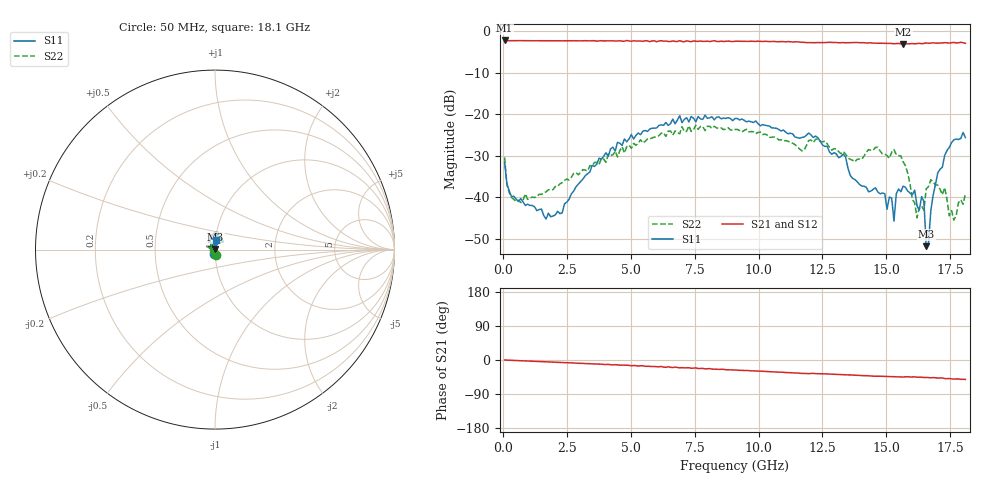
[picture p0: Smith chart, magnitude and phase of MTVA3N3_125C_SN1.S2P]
! Network Analyzer HP8720D.06.14 Serial No. US36140669
! 27 Jun 2005  08:55:49
! Frequency  S11  S21  S12  S22
# HZ  S  DB R 50
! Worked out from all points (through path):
!   201 points, 50 MHz to 18.1 GHz, reference 50 ohm
!   highest |S21| = -2.27 dB at 50 MHz (marker M1); lowest = -3.1 dB at 15.66 GHz (marker M2)
!   group delay of S21, straight-line fit = 7.91 ps
!   lowest |S11| = -51.8 dB at 16.57 GHz (marker M3), VSWR 1.01, Z = 50.2 + j0.173 ohm
!   |S11| at or under -10 dB: start of sweep to end of sweep
!   |S22| runs from -45.5 to -22.7 dB; largest |S21 - S12| = 0.022
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5e7  -31.66 -100.6  -2.27 0.1  -2.29 0.3  -30.42 -79.3
1.4025e8  -36.78 -122.5  -2.32 -0.3  -2.32 -0.2  -36.95 -115.0
5.0125e8  -40.44 -155.0  -2.33 -1.5  -2.32 -1.5  -41.04 -155.6
1.6745e9  -45.24 147.2  -2.34 -4.8  -2.34 -4.9  -38.70 161.6
3.1185e9  -35.62 79.8  -2.35 -8.9  -2.37 -9.1  -33.35 131.8
6.09675e9  -22.70 79.9  -2.41 -17.8  -2.35 -17.7  -25.16 79.4
9.075e9  -21.05 95.4  -2.47 -26.4  -2.45 -26.5  -23.70 51.4
1.21435e10  -25.63 125.2  -2.81 -35.3  -2.78 -35.5  -26.84 89.1
1.331675e10  -29.61 126.7  -2.79 -38.7  -2.81 -38.9  -29.00 111.4
1.3768e10  -35.73 137.3  -2.75 -40.2  -2.79 -40.2  -31.48 139.6
1.494125e10  -39.12 161.3  -2.95 -43.2  -3.00 -42.9  -29.60 156.5
1.50315e10  -42.91 167.3  -3.01 -43.4  -2.99 -44.0  -29.98 167.1
1.512175e10  -39.92 123.2  -3.01 -43.8  -2.96 -43.6  -30.64 166.3
1.530225e10  -45.73 94.1  -3.07 -44.0  -2.96 -44.7  -28.50 165.5
1.53925e10  -39.16 59.4  -3.03 -44.5  -2.97 -44.1  -29.78 162.1
1.566325e10  -37.30 9.3  -3.11 -45.1  -3.07 -44.3  -31.50 141.8
1.620475e10  -42.07 2.2  -3.02 -45.3  -3.02 -44.9  -44.95 18.9
1.64755e10  -41.02 18.9  -2.98 -46.1  -3.12 -45.2  -43.12 -49.7
1.656575e10  -51.77 41.9  -2.87 -46.0  -2.89 -46.3  -37.99 -53.5
1.7017e10  -34.13 98.3  -2.92 -47.8  -3.00 -48.6  -37.07 -107.5
1.764875e10  -26.17 88.6  -2.75 -50.3  -2.68 -50.4  -45.49 -129.5
1.81e10  -25.64 82.2  -2.96 -51.3  -2.94 -52.2  -39.14 -166.6
